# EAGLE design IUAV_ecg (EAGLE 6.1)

## Sheet 1 of 5: Info
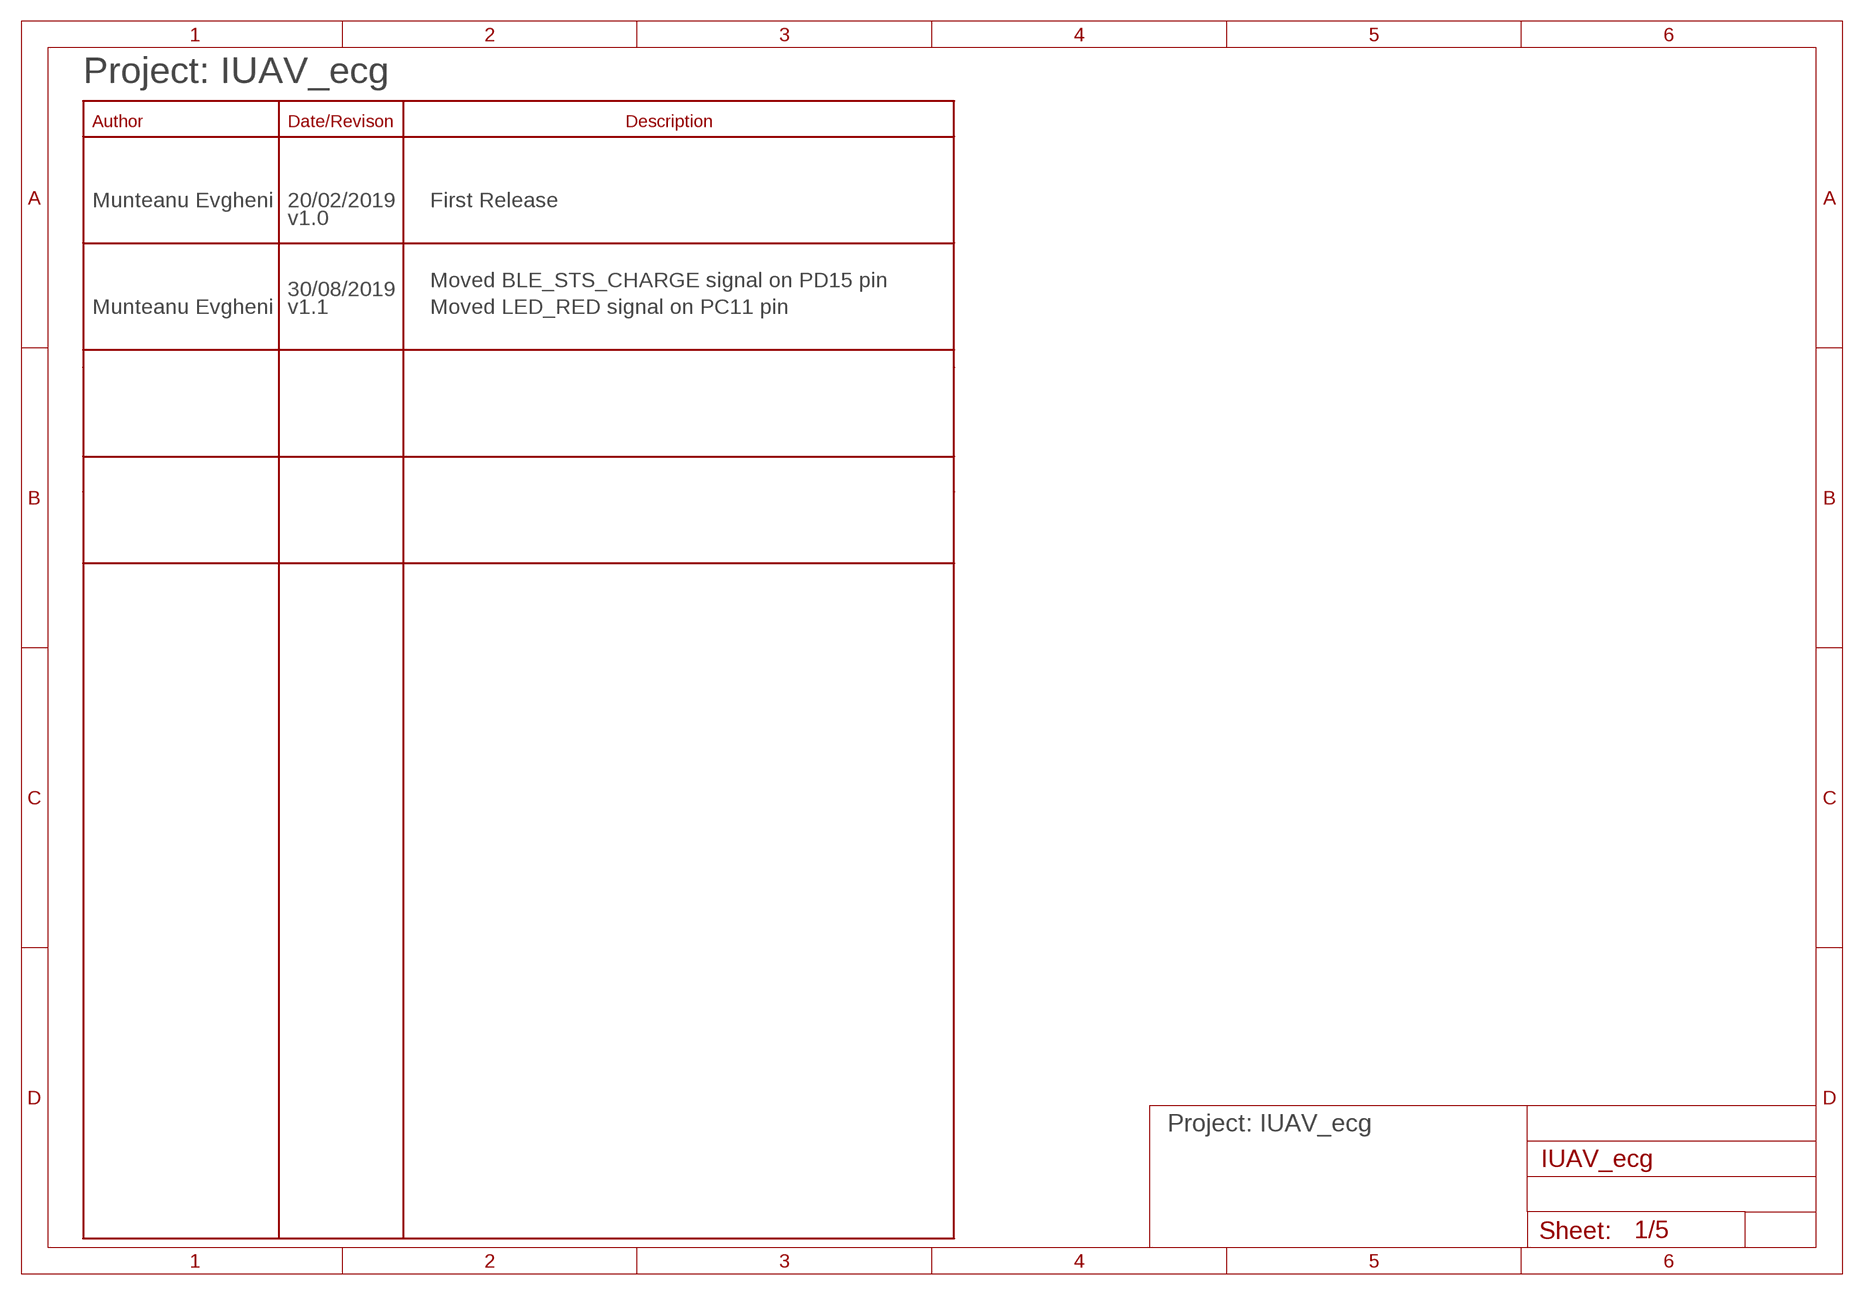
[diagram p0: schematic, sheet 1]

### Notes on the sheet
- Project: IUAV_ecg
- Munteanu Evgheni | 20/02/2019 | First Release
- v1.0
- Moved BLE_STS_CHARGE signal on PD15 pin
- 30/08/2019
- Munteanu Evgheni | v1.1 | Moved LED_RED signal on PC11 pin
- Project: IUAV_ecg

## Sheet 2 of 5: Power Management
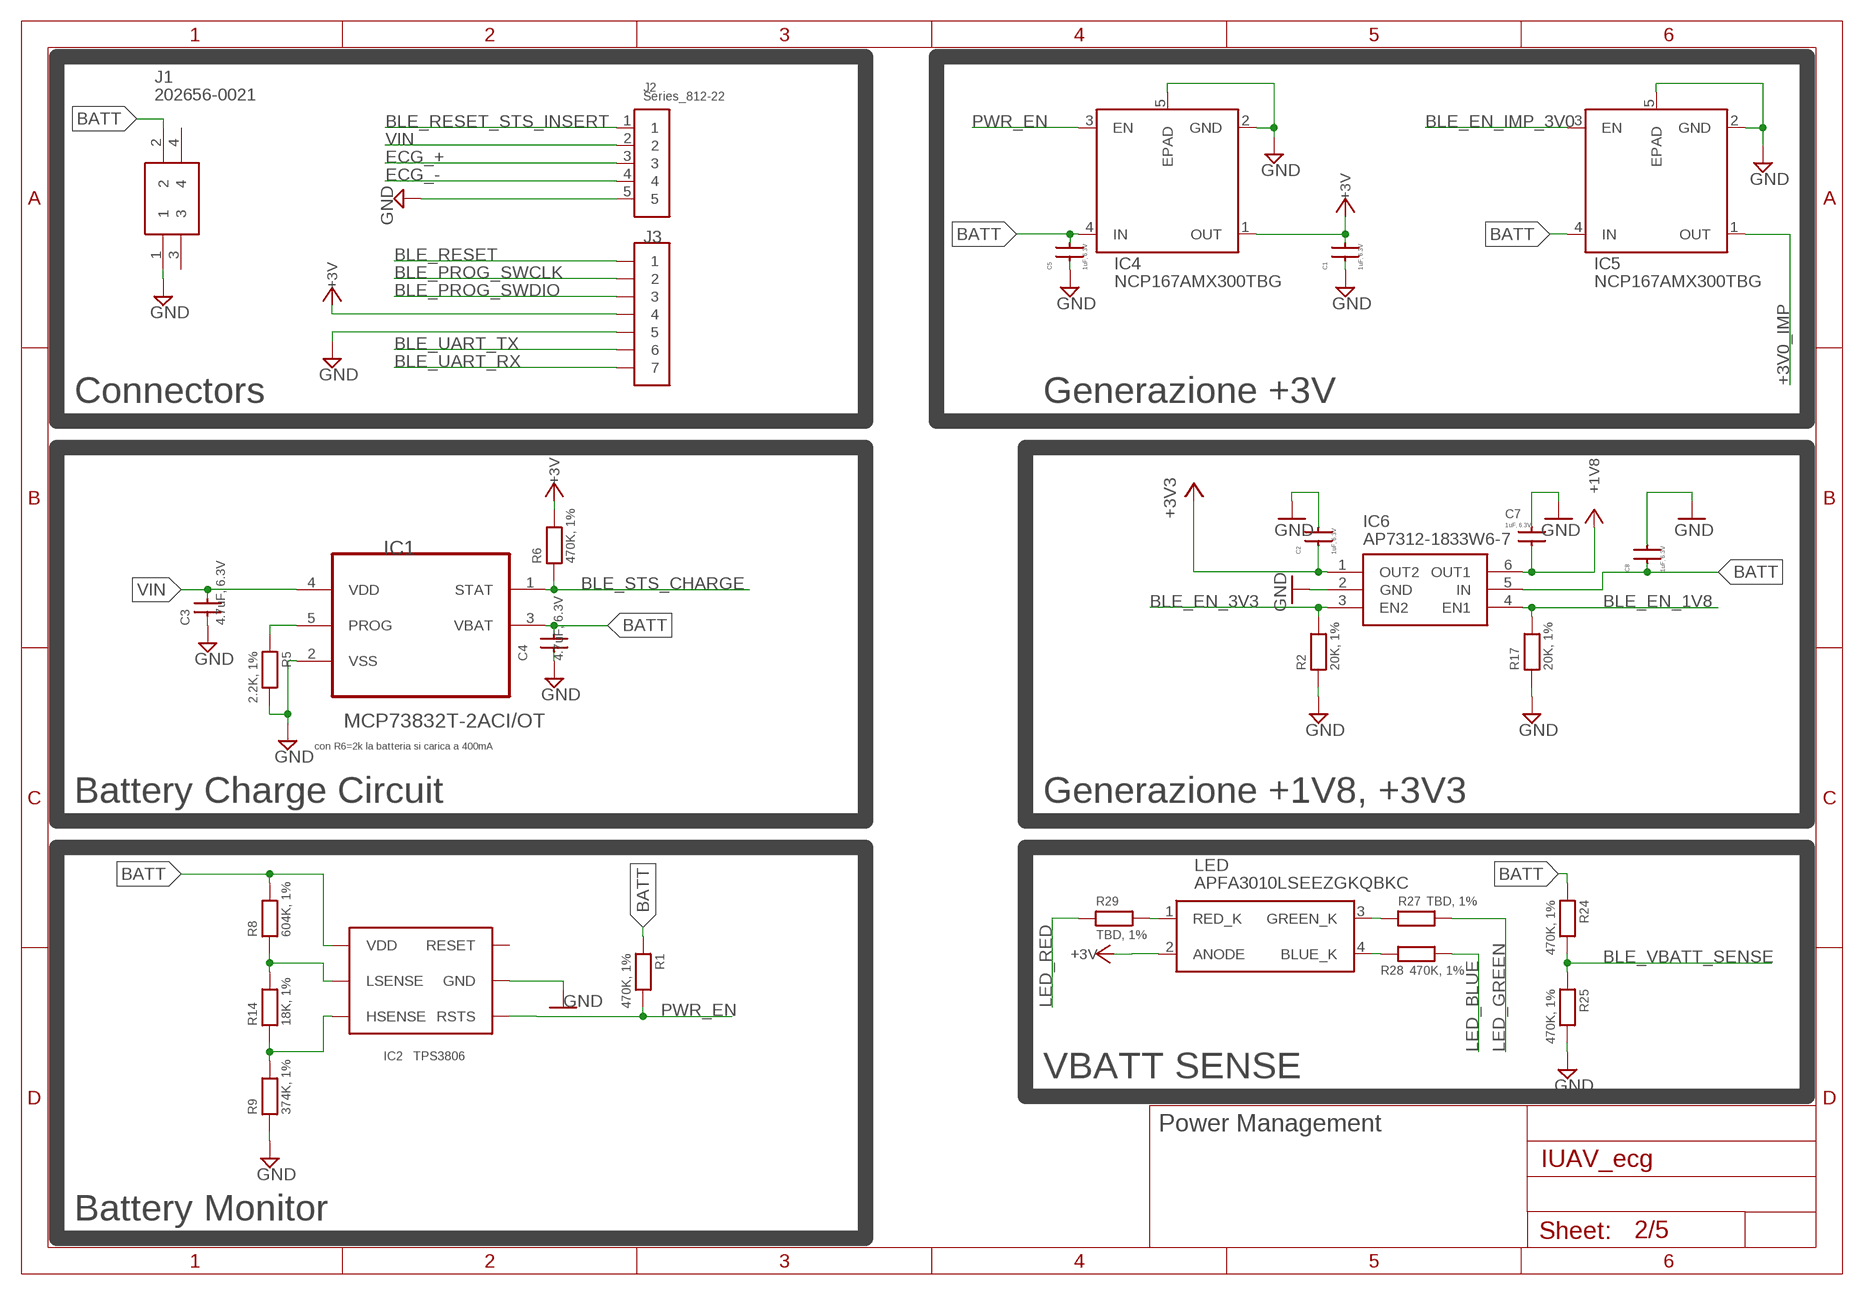
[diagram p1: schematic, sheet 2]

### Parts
C1  1uF, 6.3V  C0402  [R0402]
C2  1uF, 6.3V  C0402  [R0402]
C3  4.7uF, 6.3V  C0402  [R0402]
C4  4.7uF, 6.3V  C0402  [R0402]
C5  1uF, 6.3V  C0402  [R0402]
C7  1uF, 6.3V  C0402  [R0402]
C8  1uF, 6.3V  C0402  [R0402]
IC1  MCP73832T-2ACI/OT  MCP73831T-2ACI/OT  [SOT95P280X145-5N]
IC2  TPS3806  [SOT23_6_DBV]
IC4  NCP167AMX300TBG  NCP167  [NCP167]
IC5  NCP167AMX300TBG  NCP167  [NCP167]
IC6  AP7312-1833W6-7  [SOT95P285X145-6N]
J1  202656-0021  [2026560021]
J2  Series_812-22  CONNECTOR_MOLLA_2.54_5P  [CONNETTORE_MOLLA_2.54_5P]
J3  PINS_PROG_1.27MM_7P  [PINS_GENERIC_1.27_7P]
LED  APFA3010LSEEZGKQBKC  [KPFA-3010RGBC-11]
R1  470K, 1%  R0402  [R0402]
R2  20K, 1%  R0402  [R0402]
R5  2.2K, 1%  R0402  [R0402]
R6  470K, 1%  R0402  [R0402]
R8  604K, 1%  R0402  [R0402]
R9  374K, 1%  R0402  [R0402]
R14  18K, 1%  R0402  [R0402]
R17  20K, 1%  R0402  [R0402]
R24  470K, 1%  R0402  [R0402]
R25  470K, 1%  R0402  [R0402]
R27  TBD, 1%  R0402  [R0402]
R28  470K, 1%  R0402  [R0402]
R29  TBD, 1%  R0402  [R0402]

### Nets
+1V8: C7.P$1 IC6.6(OUT1) ; also sheet 5
+3V: C1.P$2 IC4.1(OUT) J3.4 LED.2(ANODE) R6.P$2 ; also sheet 3,5
+3V0_IMP: IC5.1(OUT) ; also sheet 4
+3V3: C2.P$1 IC6.1(OUT2) ; also sheet 5
BATT: C4.P$2 C5.P$2 C8.P$1 IC1.3(VBAT) IC2.P$4(VDD) IC4.4(IN) IC5.4(IN) IC6.5(IN) J1.2 R1.P$1 R8.P$2 R24.P$1
BLE_EN_1V8: IC6.4(EN1) R17.P$2 ; also sheet 3
BLE_EN_3V3: IC6.3(EN2) R2.P$2 ; also sheet 3
BLE_EN_IMP_3V0: IC5.3(EN) ; also sheet 3
BLE_PROG_SWCLK: J3.2 ; also sheet 3
BLE_PROG_SWDIO: J3.3 ; also sheet 3
BLE_RESET: J3.1 ; also sheet 3
BLE_RESET_STS_INSERT: J2.1 ; also sheet 3
BLE_STS_CHARGE: IC1.1(STAT) R6.P$1 ; also sheet 3
BLE_UART_RX: J3.7 ; also sheet 3
BLE_UART_TX: J3.6 ; also sheet 3
BLE_VBATT_SENSE: R24.P$2 R25.P$1 ; also sheet 3
ECG_+: J2.3 ; also sheet 5
ECG_-: J2.4 ; also sheet 5
GND: C1.P$1 C2.P$2 C3.P$1 C4.P$1 C5.P$1 C7.P$2 C8.P$2 IC1.2(VSS) IC2.P$2(GND) IC4.2(GND) IC4.5(EPAD) IC5.2(GND) IC5.5(EPAD) IC6.2(GND) J1.1 J2.5 J3.5 R2.P$1 R5.P$2 R9.P$1 R17.P$1 R25.P$2 ; also sheet 3,4,5
LED_BLUE: R28.P$1 ; also sheet 3
LED_GREEN: R27.P$2 ; also sheet 3
LED_RED: R29.P$1 ; also sheet 3
N$9: IC1.5(PROG) R5.P$1
N$11: IC2.P$5(LSENSE) R8.P$1 R14.P$2
N$13: IC2.P$6(HSENSE) R9.P$2 R14.P$1
N$17: LED.1(RED_K) R29.P$2
N$18: LED.4(BLUE_K) R28.P$2
N$19: LED.3(GREEN_K) R27.P$1
PWR_EN: IC2.P$1(RSTS) IC4.3(EN) R1.P$2
VIN: C3.P$2 IC1.4(VDD) J2.2
Unconnected: IC2.P$3(RESET) J1.3 J1.4

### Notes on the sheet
- Connectors | Generazione +3V
- con R6=2k la batteria si carica a 400mA
- Battery Charge Circuit | Generazione +1V8, +3V3
- VBATT SENSE
- Power Management
- Battery Monitor

## Sheet 3 of 5: Bluetooth
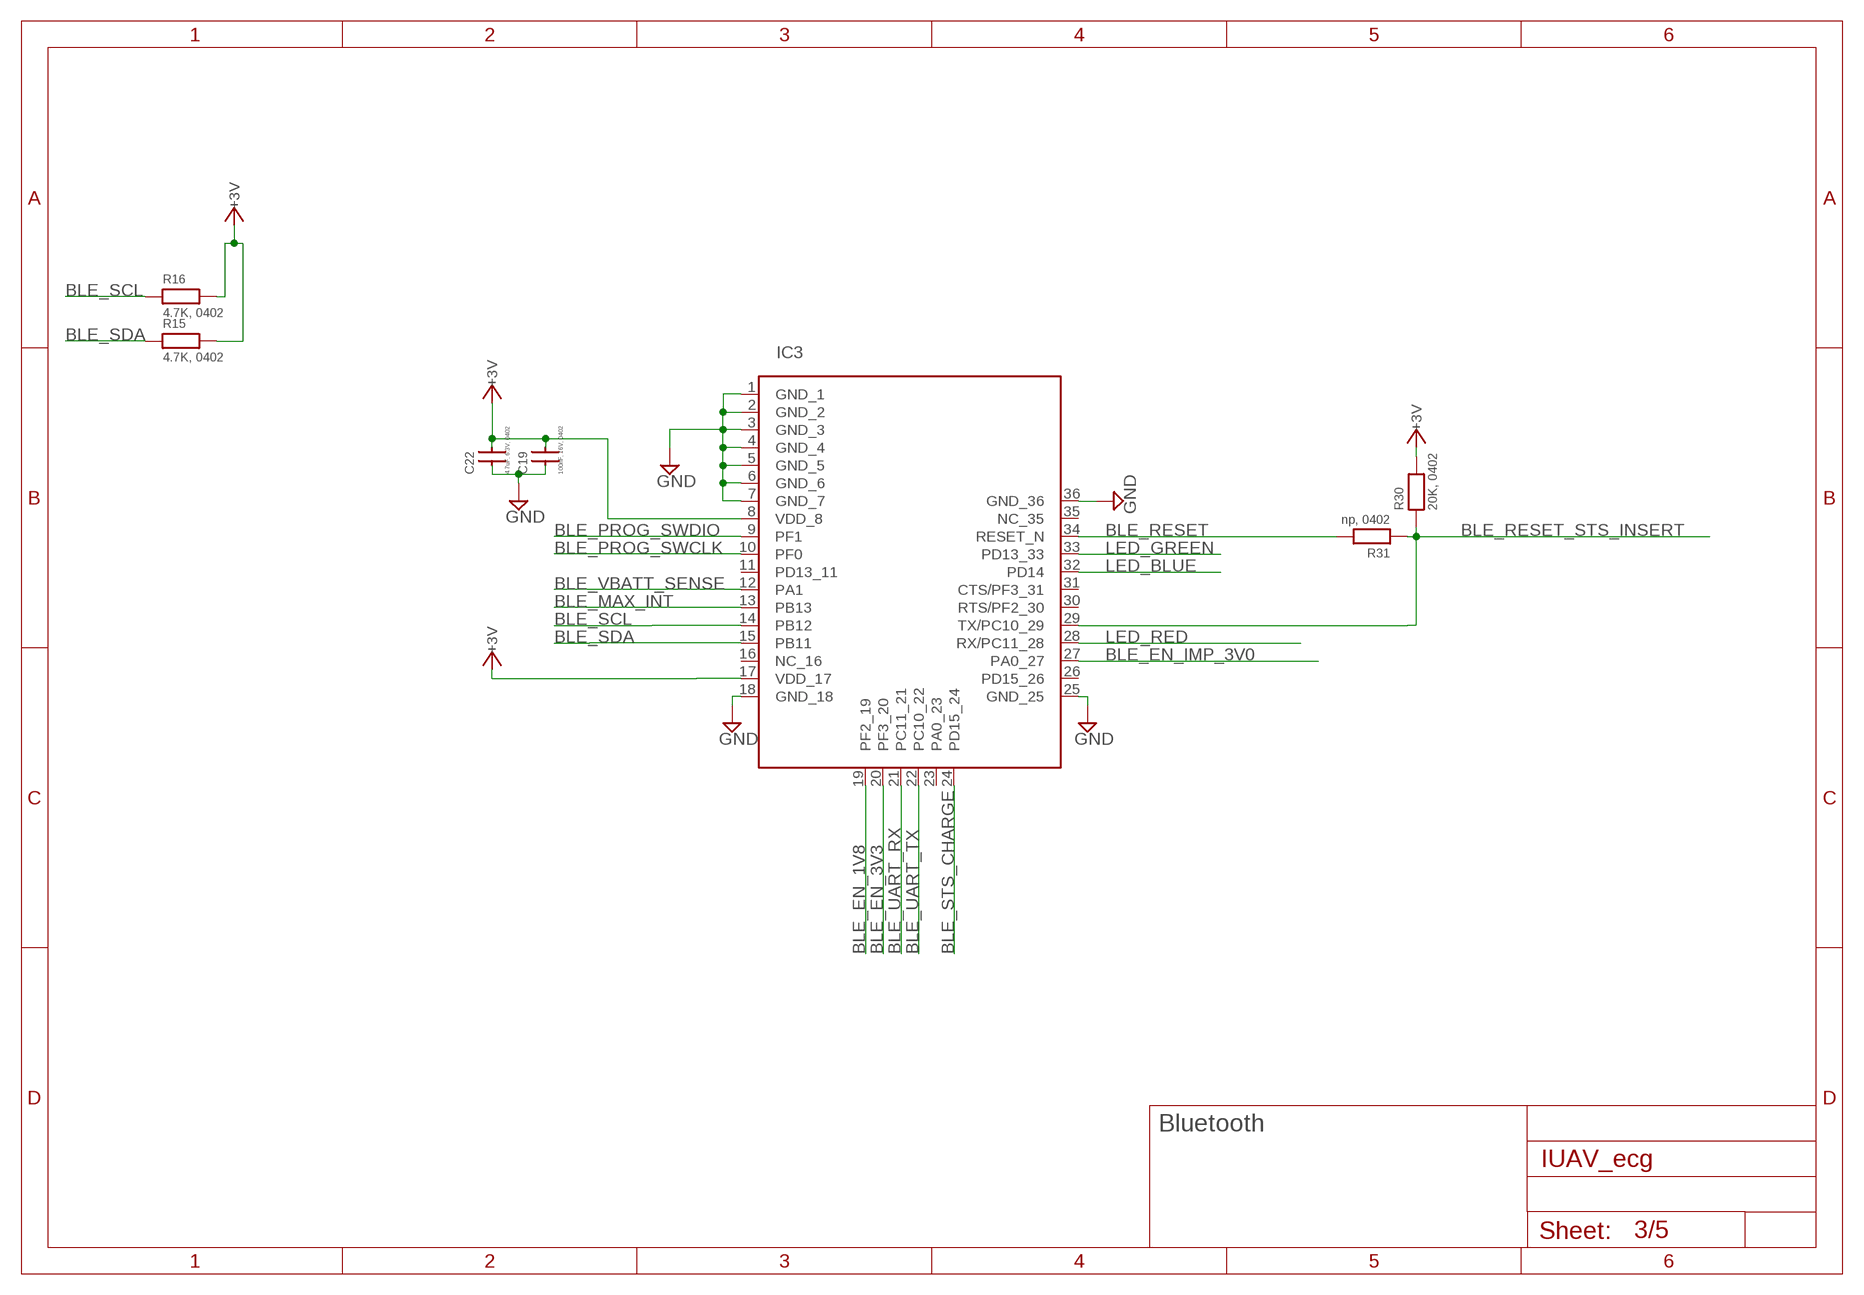
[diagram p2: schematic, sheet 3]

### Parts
C19  100nF, 16V, 0402  C0402  [R0402]
C22  4.7uF, 6.3V, 0402  C0402  [R0402]
IC3  BGM113  [BGM113]
R15  4.7K, 0402  R0402  [R0402]
R16  4.7K, 0402  R0402  [R0402]
R30  20K, 0402  R0402  [R0402]
R31  np, 0402  R0402  [R0402]

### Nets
+3V: C19.P$2 C22.P$2 IC3.8(VDD_8) IC3.17(VDD_17) R15.P$2 R16.P$2 R30.P$2 ; also sheet 2,5
BLE_EN_1V8: IC3.19(PF2_19) ; also sheet 2
BLE_EN_3V3: IC3.20(PF3_20) ; also sheet 2
BLE_EN_IMP_3V0: IC3.27(PA0_27) ; also sheet 2
BLE_MAX_INT: IC3.13(PB13) ; also sheet 5
BLE_PROG_SWCLK: IC3.10(PF0) ; also sheet 2
BLE_PROG_SWDIO: IC3.9(PF1) ; also sheet 2
BLE_RESET: IC3.34(RESET_N) R31.P$2 ; also sheet 2
BLE_RESET_STS_INSERT: IC3.29(TX/PC10_29) R30.P$1 R31.P$1 ; also sheet 2
BLE_SCL: IC3.14(PB12) R16.P$1 ; also sheet 4,5
BLE_SDA: IC3.15(PB11) R15.P$1 ; also sheet 4,5
BLE_STS_CHARGE: IC3.24(PD15_24) ; also sheet 2
BLE_UART_RX: IC3.21(PC11_21) ; also sheet 2
BLE_UART_TX: IC3.22(PC10_22) ; also sheet 2
BLE_VBATT_SENSE: IC3.12(PA1) ; also sheet 2
GND: C19.P$1 C22.P$1 IC3.1(GND_1) IC3.2(GND_2) IC3.3(GND_3) IC3.4(GND_4) IC3.5(GND_5) IC3.6(GND_6) IC3.7(GND_7) IC3.18(GND_18) IC3.25(GND_25) IC3.36(GND_36) ; also sheet 2,4,5
LED_BLUE: IC3.32(PD14) ; also sheet 2
LED_GREEN: IC3.33(PD13_33) ; also sheet 2
LED_RED: IC3.28(RX/PC11_28) ; also sheet 2
Unconnected: IC3.11(PD13_11) IC3.16(NC_16) IC3.23(PA0_23) IC3.26(PD15_26) IC3.30(RTS/PF2_30) IC3.31(CTS/PF3_31) IC3.35(NC_35)

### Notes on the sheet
- Bluetooth

## Sheet 4 of 5: Sensore Impedenza
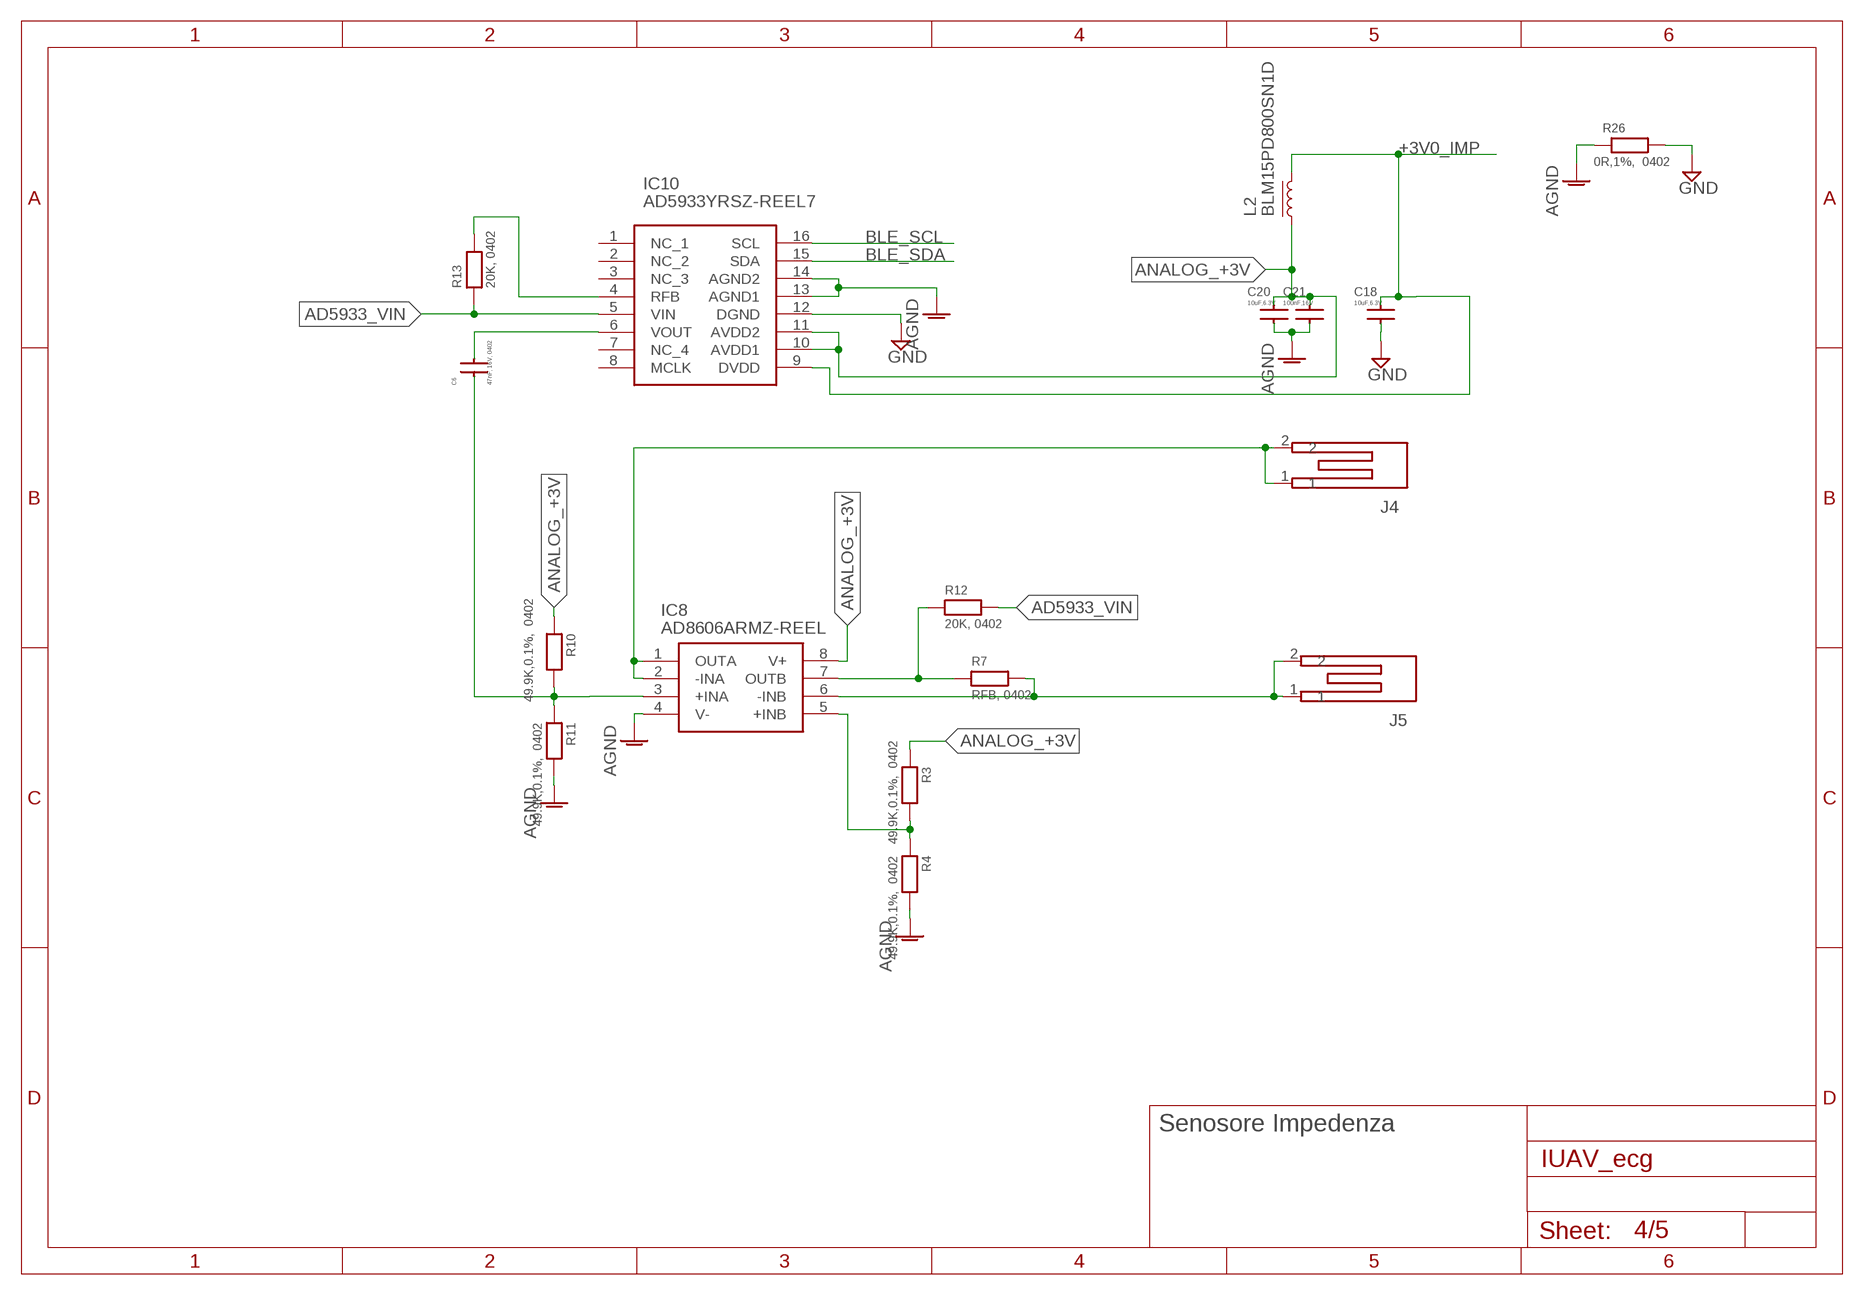
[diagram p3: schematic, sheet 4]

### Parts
C6  47nF, 16V, 0402  C0402  [R0402]
C18  10uF,6.3V  C0402  [R0402]
C20  10uF,6.3V  C0402  [R0402]
C21  100nF,16V  C0402  [R0402]
IC8  AD8606ARMZ-REEL  [SOP65P490X110-8N]
IC10  AD5933YRSZ-REEL7  [SOP65P780X200-16N]
J4  CONTACT_2040852-1  [CONTACT_2040852-1]
J5  CONTACT_2040852-1  [CONTACT_2040852-1]
L2  BLM15PD800SN1D  INDUTTORE_FILTRO  [SMD_0402]
R3  49.9K,0.1%, 0402  R0402  [R0402]
R4  49.9K,0.1%, 0402  R0402  [R0402]
R7  RFB, 0402  R0402  [R0402]
R10  49.9K,0.1%, 0402  R0402  [R0402]
R11  49.9K,0.1%, 0402  R0402  [R0402]
R12  20K, 0402  R0402  [R0402]
R13  20K, 0402  R0402  [R0402]
R26  0R,1%, 0402  R0402  [R0402]

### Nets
+3V0_IMP: C18.P$2 IC10.9(DVDD) L2.P$2 ; also sheet 2
AD5933_VIN: IC10.5(VIN) R12.P$2 R13.P$1
AGND: C20.P$1 C21.P$1 IC8.4(V-) IC10.13(AGND1) IC10.14(AGND2) R4.P$2 R11.P$2 R26.P$1
ANALOG_+3V: C20.P$2 C21.P$2 IC8.8(V+) IC10.10(AVDD1) IC10.11(AVDD2) L2.P$1 R3.P$1 R10.P$1
BLE_SCL: IC10.16(SCL) ; also sheet 3,5
BLE_SDA: IC10.15(SDA) ; also sheet 3,5
GND: C18.P$1 IC10.12(DGND) R26.P$2 ; also sheet 2,3,5
N$4: IC8.5(+INB) R3.P$2 R4.P$1
N$5: IC8.7(OUTB) R7.P$1 R12.P$1
N$6: IC8.6(-INB) J5.1 J5.2 R7.P$2
N$8: C6.P$2 IC10.6(VOUT)
N$10: C6.P$1 IC8.3(+INA) R10.P$2 R11.P$1
N$14: IC8.1(OUTA) IC8.2(-INA) J4.1 J4.2
N$16: IC10.4(RFB) R13.P$2
Unconnected: IC10.1(NC_1) IC10.2(NC_2) IC10.3(NC_3) IC10.7(NC_4) IC10.8(MCLK)

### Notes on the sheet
- Senosore Impedenza

## Sheet 5 of 5: Sensore ECG
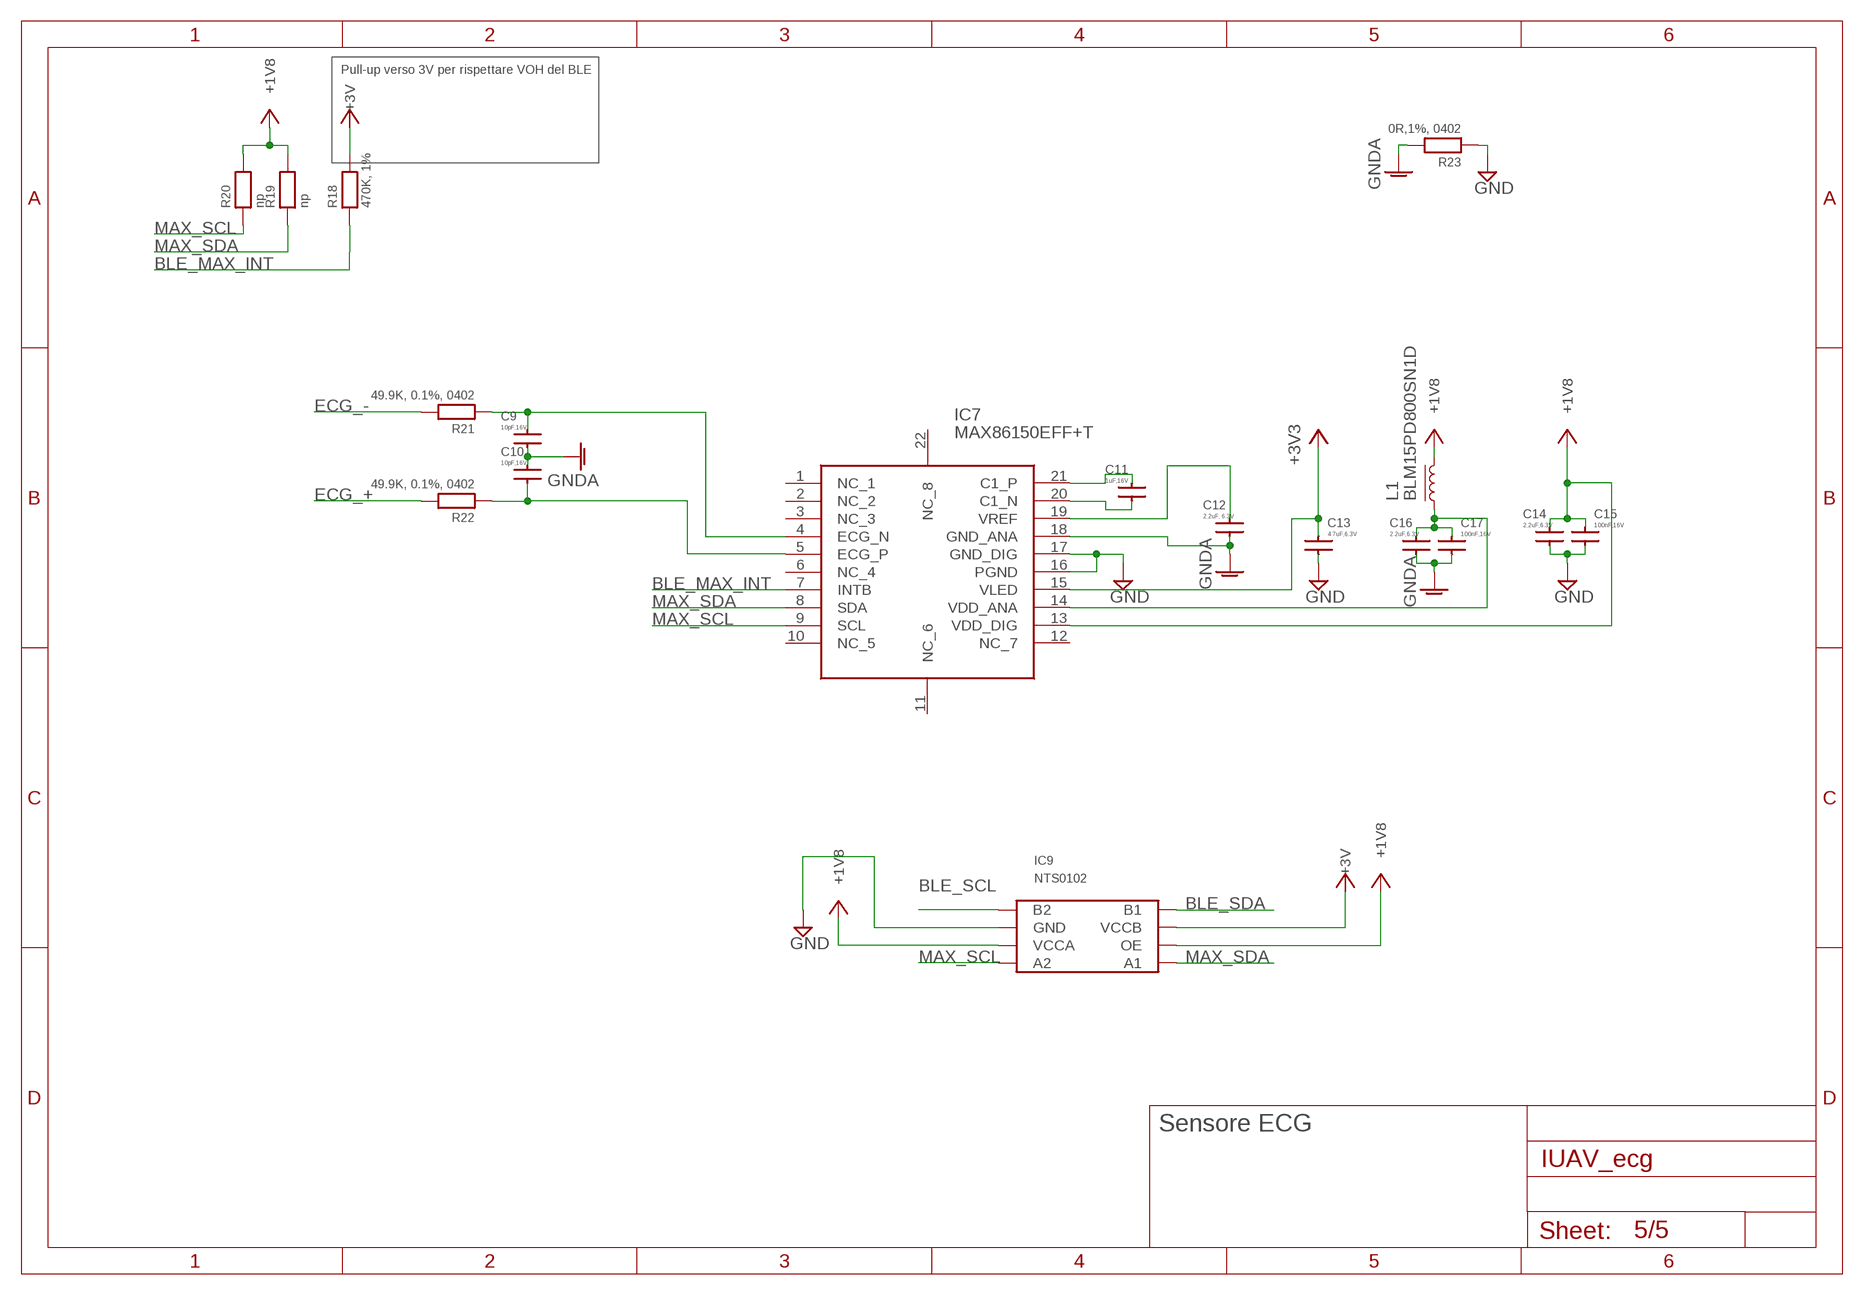
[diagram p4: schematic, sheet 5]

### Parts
C9  10pF,16V  C0402  [R0402]
C10  10pF,16V  C0402  [R0402]
C11  1uF,16V  C0402  [R0402]
C12  2.2uF, 6.3V  C0402  [R0402]
C13  4.7uF,6.3V  C0402  [R0402]
C14  2.2uF,6.3V  C0402  [R0402]
C15  100nF,16V  C0402  [R0402]
C16  2.2uF,6.3V  C0402  [R0402]
C17  100nF,16V  C0402  [R0402]
IC7  MAX86150EFF+T  [MAX86150EFFT]
IC9  NTS0102  [SOT996-2]
L1  BLM15PD800SN1D  INDUTTORE_FILTRO  [SMD_0402]
R18  470K, 1%  R0402  [R0402]
R19  np  R0402  [R0402]
R20  np  R0402  [R0402]
R21  49.9K, 0.1%, 0402  R0402  [R0402]
R22  49.9K, 0.1%, 0402  R0402  [R0402]
R23  0R,1%, 0402  R0402  [R0402]

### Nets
+1V8: C14.P$2 C15.P$2 IC7.13(VDD_DIG) IC9.3(VCCA) IC9.6(OE) L1.P$2 R19.P$2 R20.P$2 ; also sheet 2
+3V: IC9.7(VCCB) R18.P$2 ; also sheet 2,3
+3V3: C13.P$2 IC7.15(VLED) ; also sheet 2
BLE_MAX_INT: IC7.7(INTB) R18.P$1 ; also sheet 3
BLE_SCL: IC9.1(B2) ; also sheet 3,4
BLE_SDA: IC9.8(B1) ; also sheet 3,4
ECG_+: R22.P$2 ; also sheet 2
ECG_-: R21.P$2 ; also sheet 2
GND: C13.P$1 C14.P$1 C15.P$1 IC7.16(PGND) IC7.17(GND_DIG) IC9.2(GND) R23.P$1 ; also sheet 2,3,4
GNDA: C9.P$1 C10.P$2 C12.P$1 C16.P$1 C17.P$1 IC7.18(GND_ANA) R23.P$2
MAX_SCL: IC7.9(SCL) IC9.4(A2) R20.P$1
MAX_SDA: IC7.8(SDA) IC9.5(A1) R19.P$1
N$1: C9.P$2 IC7.4(ECG_N) R21.P$1
N$2: C11.P$2 IC7.21(C1_P)
N$3: C10.P$1 IC7.5(ECG_P) R22.P$1
N$7: C11.P$1 IC7.20(C1_N)
N$12: C12.P$2 IC7.19(VREF)
N$15: C16.P$2 C17.P$2 IC7.14(VDD_ANA) L1.P$1
Unconnected: IC7.1(NC_1) IC7.2(NC_2) IC7.3(NC_3) IC7.6(NC_4) IC7.10(NC_5) IC7.11(NC_6) IC7.12(NC_7) IC7.22(NC_8)

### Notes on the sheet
- Pull-up verso 3V per rispettare VOH del BLE
- Sensore ECG

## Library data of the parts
C1-C22 = VIBRAM_LIB:C0402
IC1 = vibram:MCP73831T-2ACI/OT: Charge Management Controller; MPN: MCP73831T-2ACI/OT; OC_FARNELL: 1332158; OC_NEWARK: 56K7045; PACKAGE: SOT-5; SUPPLIER: Microchip
IC2 = VIBRAM_LIB:TPS3806
IC3 = RELab_ElectronicLibrary:BGM113
IC4 IC5 = RELab_ElectronicLibrary:NCP167
IC6 = SamacSys_Parts:AP7312-1833W6-7: LDO,Regulator,Pos,reg,3.3V,0.15A,SOT26 DiodesZetex AP7312-1833W6-7, Dual LDO Voltage Regulator, 150mA, 1.8 V, 3.3 V /-2%, 6-Pin SOT-26 Source: Datasheet; DESCRIPTION: LDO,Regulator,Pos,reg,3.3V,0.15A,SOT26 DiodesZetex AP7312-1833W6-7, Dual LDO Voltage Regulator, 150mA, 1.8 V, 3.3 V /-2%, 6-Pin SOT-26; HEIGHT: 1.45mm; MANUFACTURER_NAME: Diodes Inc.; MANUFACTURER_PART_NUMBER: AP7312-1833W6-7; MOUSER_PART_NUMBER: 621-AP7312-1833W6-7; MOUSER_PRICE-STOCK: https://www.mouser.com/Search/Refine.aspx?Keyword=621-AP7312-1833W6-7
IC7 = SamacSys_Parts:MAX86150EFF+T: Biometric Sensors Pulse Oximetry/Heart Rate Bio Sensor Source: Datasheet; DESCRIPTION: Biometric Sensors Pulse Oximetry/Heart Rate Bio Sensor; HEIGHT: 1.4mm; MANUFACTURER_NAME: Maxim Integrated; MANUFACTURER_PART_NUMBER: MAX86150EFF+T; MOUSER_PART_NUMBER: 700-MAX86150EFF+T; MOUSER_PRICE-STOCK: https://www.mouser.com/Search/Refine.aspx?Keyword=700-MAX86150EFF%2BT
IC8 = SamacSys_Parts:AD8606ARMZ-REEL: Precision, Low Noise, CMOS, Rail-to-Rail,%D Input/Output Operational Amplifiers Source: Datasheet; DESCRIPTION: Precision, Low Noise, CMOS, Rail-to-Rail,%D Input/Output Operational Amplifiers; HEIGHT: 1.1mm; MANUFACTURER_NAME: Analog Devices; MANUFACTURER_PART_NUMBER: AD8606ARMZ-REEL; MOUSER_PART_NUMBER: 584-AD8606ARMZ-R; MOUSER_PRICE-STOCK: https://www.mouser.com/Search/Refine.aspx?Keyword=584-AD8606ARMZ-R
IC9 = RELab_ElectronicLibrary:NTS0102
IC10 = SamacSys_Parts:AD5933YRSZ-REEL7: Data Acquisition ADCs/DACs - Specialized IC 12bit 1 MSPS Impedance Cnvtr Source: Datasheet; DESCRIPTION: Data Acquisition ADCs/DACs - Specialized IC 12bit 1 MSPS Impedance Cnvtr; HEIGHT: 2mm; MANUFACTURER_NAME: Analog Devices; MANUFACTURER_PART_NUMBER: AD5933YRSZ-REEL7; MOUSER_PART_NUMBER: 584-AD5933YRSZ-R7; MOUSER_PRICE-STOCK: https://www.mouser.com/Search/Refine.aspx?Keyword=584-AD5933YRSZ-R7
J1 = SamacSys_Parts:202656-0021: MOLEX - 202656-0021 - PLUG HOUSING, 2POS, NYLON, BLACK Source: Datasheet; DESCRIPTION: MOLEX - 202656-0021 - PLUG HOUSING, 2POS, NYLON, BLACK; HEIGHT: 1mm; MANUFACTURER_NAME: Molex; MANUFACTURER_PART_NUMBER: 202656-0021; MOUSER_PART_NUMBER: 538-202656-0021; MOUSER_PRICE-STOCK: https://www.mouser.com/Search/Refine.aspx?Keyword=538-202656-0021
J2 = RELab_ElectronicLibrary:CONNECTOR_MOLLA_2.54_5P
J3 = RELab_ElectronicLibrary:PINS_PROG_1.27MM_7P
J4 J5 = RELab_ElectronicLibrary:CONTACT_2040852-1
L1 L2 = RELab_ElectronicLibrary:INDUTTORE_FILTRO
LED = SamacSys_Parts:APFA3010LSEEZGKQBKC: 3.0x1.0mm RIGHT ANGLE SMD CHIP LED LAMP Source: Datasheet; DESCRIPTION: 3.0x1.0mm RIGHT ANGLE SMD CHIP LED LAMP; HEIGHT: mm; MANUFACTURER_NAME: Kingbright; MANUFACTURER_PART_NUMBER: APFA3010LSEEZGKQBKC; MOUSER_PART_NUMBER: 604-APFA3010LSEEZGKQ; MOUSER_PRICE-STOCK: https://www.mouser.com/Search/Refine.aspx?Keyword=604-APFA3010LSEEZGKQ
R1-R31 = VIBRAM_LIB:R0402

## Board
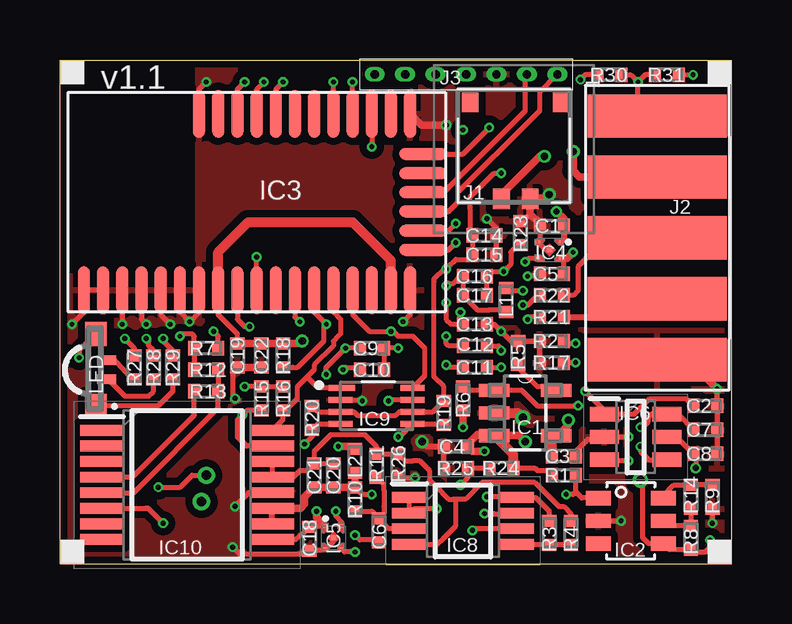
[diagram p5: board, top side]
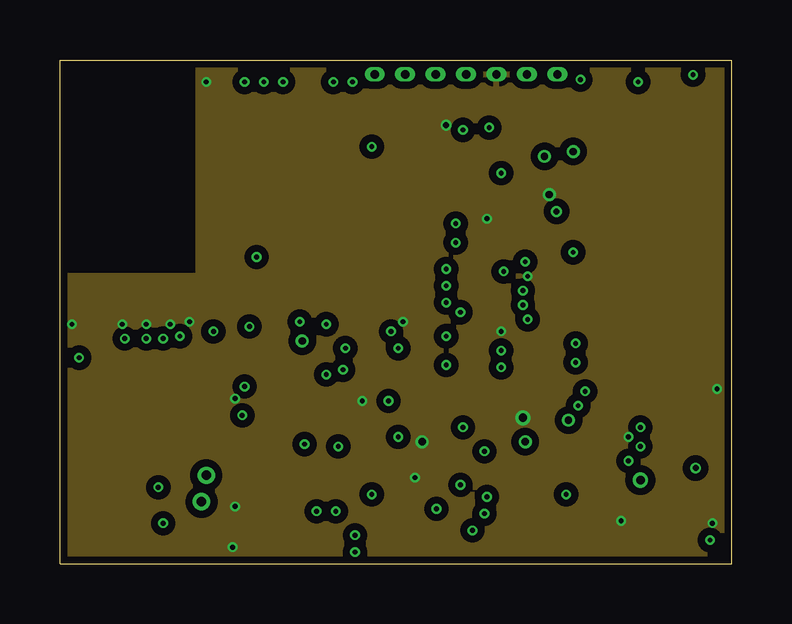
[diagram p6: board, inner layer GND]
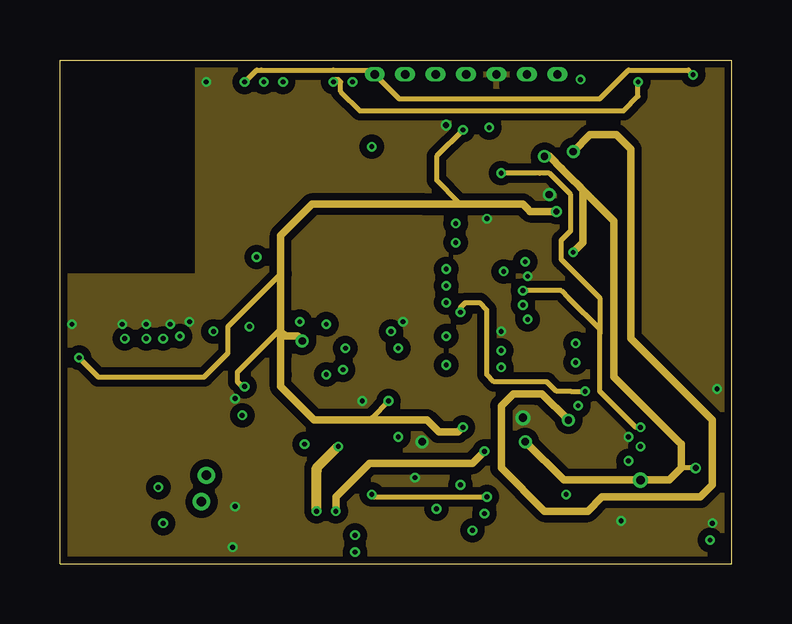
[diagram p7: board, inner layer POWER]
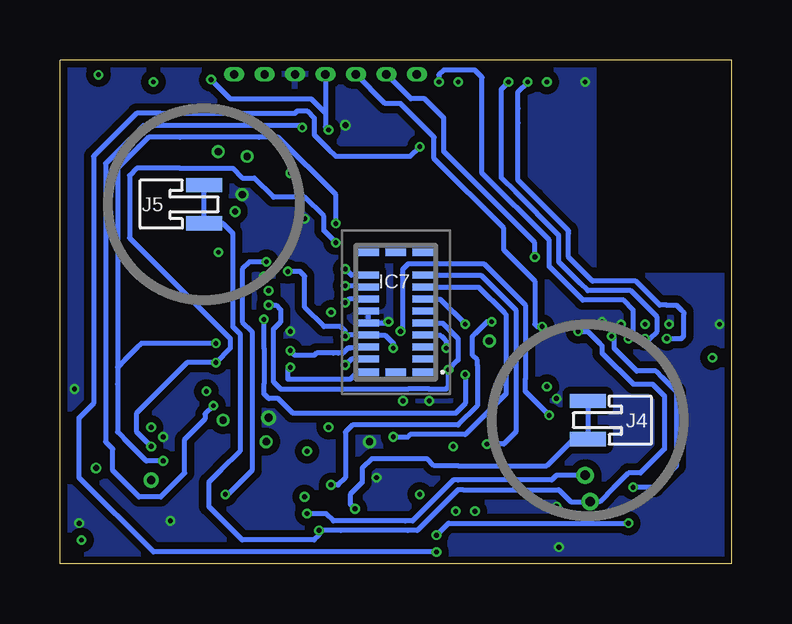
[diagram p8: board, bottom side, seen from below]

Size 28 x 21 mm. Coordinates in mm from the lower left corner, seen from the top.
Outline: 28,0 28,21 0,21 0,0 28,0
Copper layers (1+2*3+16): Top 0.035mm / dielectric 0.38mm / GND 0.035mm / dielectric 0.71mm / POWER 0.035mm / dielectric 0.38mm / Bottom 0.035mm
Design rules: minimum track width 0.2mm, minimum drill 0.2mm, track to track 0.2mm, track to pad 0.2mm, pad to pad 0.2mm, via to via 0.2mm, smd to smd 0.15mm, copper to edge 0.2mm, drill to drill 0.2mm, minimum pad ring 0.1mm, minimum via ring 0.1mm, stop-mask expansion 0.075mm, vias tented up to drill 12mil, thermal gap 0.2mm

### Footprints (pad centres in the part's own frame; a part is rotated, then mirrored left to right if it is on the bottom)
R0402 = smd 0.5 x 0.6: P$1 -0.5,0; P$2 0.5,0
SOT95P280X145-5N = smd 1.27 x 0.559: 1 -1.295,0.94; 2 -1.295,0; 3 -1.295,-0.94; 4 1.295,-0.94; 5 1.295,0.94
SOT23_6_DBV = smd 0.6 x 1.05: P$1 -0.95,-1.35; P$2 0,-1.35; P$3 0.95,-1.35; P$4 0.95,1.35; P$5 0,1.35; P$6 -0.95,1.35
BGM113 = smd 2 x 0.5: 1 -3.675,7.2; 2 -3.675,6.4; 3 -3.675,5.6; 4 -3.675,4.8; 5 -3.675,4; 6 -3.675,3.2; 7 -3.675,2.4; 8 -3.675,1.6; 9 -3.675,0.8; 10 -3.675,0; 11 -3.675,-0.8; 12 -3.675,-1.6; 13 -3.675,-2.4; 14 -3.675,-3.2; 15 -3.675,-4; 16 -3.675,-4.8; 17 -3.675,-5.6; 18 -3.675,-6.4; 25 3.675,-6.4; 26 3.675,-5.6; 27 3.675,-4.8; 28 3.675,-4; 29 3.675,-3.2; 30 3.675,-2.4; 31 3.675,-1.6; 32 3.675,-0.8; 33 3.675,0; 34 3.675,0.8; 35 3.675,1.6; 36 3.675,2.4 | smd 0.5 x 2: 19 -2,-6.95; 20 -1.2,-6.95; 21 -0.4,-6.95; 22 0.4,-6.95; 23 1.2,-6.95; 24 2,-6.95
NCP167 = smd 0.2 x 0.2: 1 -0.355,0.5; 2 -0.355,-0.5; 3 0.355,-0.5; 4 0.355,0.5; 5 0,0
SOT95P285X145-6N = smd 1.2 x 0.6: 1 -1.3,0.95; 2 -1.3,0; 3 -1.3,-0.95; 4 1.3,-0.95; 5 1.3,0; 6 1.3,0.95
MAX86150EFFT = smd 0.9 x 0.3: 1 -1.15,2.5; 2 -1.15,1.95; 3 -1.15,1.45; 4 -1.15,0.95; 5 -1.15,0.45; 6 -1.15,-0.05; 7 -1.15,-0.55; 8 -1.15,-1.05; 9 -1.15,-1.55; 10 -1.15,-2.5; 12 1.15,-2.5; 13 1.15,-1.55; 14 1.15,-1.05; 15 1.15,-0.55; 16 1.15,-0.05; 17 1.15,0.45; 18 1.15,0.95; 19 1.15,1.45; 20 1.15,1.95; 21 1.15,2.5 | smd 0.85 x 0.3: 11 0,-2.5; 22 0,2.5
SOP65P490X110-8N = smd 1.45 x 0.45: 1 -2.225,0.975; 2 -2.225,0.325; 3 -2.225,-0.325; 4 -2.225,-0.975; 5 2.225,-0.975; 6 2.225,-0.325; 7 2.225,0.325; 8 2.225,0.975
SOT996-2 = smd 0.25 x 1.1: 1 -0.75,-1.45 | smd 0.25 x 1: 2 -0.25,-1.5; 3 0.25,-1.5; 4 0.75,-1.5; 5 0.75,1.5; 6 0.25,1.5; 7 -0.25,1.5; 8 -0.75,1.5
SOP65P780X200-16N = smd 1.8 x 0.45: 1 -3.55,2.275; 2 -3.55,1.625; 3 -3.55,0.975; 4 -3.55,0.325; 5 -3.55,-0.325; 6 -3.55,-0.975; 7 -3.55,-1.625; 8 -3.55,-2.275; 9 3.55,-2.275; 10 3.55,-1.625; 11 3.55,-0.975; 12 3.55,-0.325; 13 3.55,0.325; 14 3.55,0.975; 15 3.55,1.625; 16 3.55,2.275
2026560021 = smd 0.7 x 0.85: 1 -0.6,2.072; 2 0.6,2.072 | smd 0.7 x 0.8: 3 -1.9,-1.953; 4 1.9,-1.953
CONNETTORE_MOLLA_2.54_5P = smd 1.8 x 5.8: 1 -5.08,0; 2 -2.54,0; 3 0,0; 4 2.54,0; 5 5.08,0
PINS_GENERIC_1.27_7P = drill 0.35 pad 0.6 long: 1 -3.81,0; 2 -2.54,0; 3 -1.27,0; 4 0,0; 5 1.27,0; 6 2.54,0; 7 3.81,0
CONTACT_2040852-1 = smd 1.5 x 0.6: 1 0,0.8; 2 0,-0.8
SMD_0402 = smd 0.5 x 0.6: P$1 -0.5,0; P$2 0.5,0
KPFA-3010RGBC-11 = smd 1 x 0.9: 1 1.5,-0.2; 2 -1.5,-0.2 | smd 0.4 x 0.8: 3 -0.4,0.25; 4 0.4,0.25

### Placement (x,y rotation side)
C1  20.5,14.1 0 top
C2  26.9,6.6 0 top
C3  21,4.5 180 top
C4  16.5,4.9 0 top
C5  20.5,12.1 0 top
C6  13.3,1.4 270 top
C7  26.9,5.6 0 top
C8  26.9,4.6 0 top
C9  13,9 180 top
C10  13,8.1 0 top
C11  17.3,8.2 0 top
C12  17.3,9.1 0 top
C13  17.3,10 180 top
C14  17.7,13.7 180 top
C15  17.7,12.9 180 top
C16  17.3,12 180 top
C17  17.3,11.2 180 top
C18  10.4,1.05 90 top
C19  7.4,8.7 90 top
C20  11.4,3.7 270 top
C21  10.6,3.7 270 top
C22  8.4,8.7 90 top
IC1  19.4,6.3 0 top
IC2  23.8,1.8 270 top
IC3  8.2,15.1 90 top
IC4  20.4,13.1 270 top
IC5  11.4,1.1 0 top
IC6  24,5.3 0 top
IC7  14,10.5 180 bottom
IC8  16.8,1.8 0 top
IC9  13.2,6.6 270 top
IC10  5.3,3.3 0 top
J1  19,17.3 180 top
J2  24.9,13.6 270 top
J3  16.93,20.42 0 top
J4  6,6 180 bottom
J5  22,15 0 bottom
L1  18.6,11 90 top
L2  12.3,4.3 90 top
LED  1.7,8.1 270 top
R1  21,3.7 0 top
R2  20.5,9.3 0 top
R3  20.4,1.3 270 top
R4  21.3,1.3 90 top
R5  19.1,8.8 90 top
R6  16.8,6.9 270 top
R7  6.1,9 0 top
R8  26.3,1.1 270 top
R9  27.2,2.8 90 top
R10  12.3,2.7 270 top
R11  13.2,4.1 90 top
R12  6.1,8.1 0 top
R13  6.1,7.2 180 top
R14  26.3,2.8 270 top
R15  8.4,6.9 90 top
R16  9.3,6.9 90 top
R17  20.5,8.4 0 top
R18  9.3,8.7 90 top
R19  16,6.3 90 top
R20  10.5,6.1 90 top
R21  20.5,10.3 0 top
R22  20.5,11.2 0 top
R23  19.2,13.8 270 top
R24  18.4,4 180 top
R25  16.5,4 180 top
R26  14.1,4.1 270 top
R27  3.1,8.2 90 top
R28  3.9,8.2 270 top
R29  4.7,8.2 270 top
R30  22.9,20.4 180 top
R31  25.3,20.4 0 top

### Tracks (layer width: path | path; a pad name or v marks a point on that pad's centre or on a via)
+1V8  (via drill 0.2)
  Top 0.2: C7.P$1 25.75,6.25 IC6.6 24.65,6.25 24.5,6.1 24.5,5.9 24.3,5.7 v24.2,5.7 | L1.P$2 18.7,11.4 v19.3,11.4 | R20.P$2 10.75,6.35 IC9.3 12.25,6.35 12.4,6.2 14,6.2 14.1,6.3 14.15,6.35 IC9.6 15.2,6.35 15.55,6.35 R19.P$2 16,7.4 15.6,7.8 15.6,11.8 15.6,11.9 16,12.3 v16.1,12.3 16.3,12.5 16.4,12.6 16.5,12.7 17,12.7 C15.P$2 C14.P$2 17.1,13.8 17.1,14.8 17.1,14.9 17.1,15.3 18.1,16.3 v18.4,16.3
  POWER 0.2: v24.2,5.7 24,5.7 23.9,5.8 22.5,7.2 22.5,7.6 22.5,7.8 22.5,9.6 | 22.5,9.6 22.5,9.8 21.2,11.1 20.9,11.4 v19.3,11.4 | v18.4,16.3 20,16.3 20.4,16.3 20.7,16 21.2,15.5 21.3,15.4 21.3,13.9 21.2,13.8 20.9,13.5 20.9,12.7 21,12.6 21.4,12.2 22.5,11.1 22.5,9.6
  Bottom 0.2: IC7.13 15.85,12.05 v16.1,12.3
+3V  (via drill 0.2, 0.25, 0.3)
  Top 0.2: R16.P$2 R15.P$2 v7.7,7.4 | IC9.7 13.75,6.85 v13.7,6.8 | LED.2 0.8,8.9 v0.8,8.6 | R30.P$2 21.9,20.4 v21.7,20.2 | C19.P$2 7.4,9.6 7.1,9.9 6.6,10.4 IC3.8
  Top 0.254: C1.P$2 21,13.55 IC4.1
  Top 0.305: C1.P$2 21,14.4 v20.7,14.7 | C19.P$2 C22.P$2 R18.P$2 10,9.2 v10.1,9.3 | R6.P$2 v16.8,5.7
  Top 0.406: IC3.8 6.6,13 7.85,14.25 12.2,14.25 13.8,12.65 IC3.17
  POWER 0.2: v7.7,7.4 7.6,7.4 7.4,7.6 7.4,8 9.2,9.8 9.2,10.2 | v13.7,6.8 13,6.1 13,6 | v16.8,18.1 15.7,17 15.7,16 16.6,15.1 16.6,15 | v0.8,8.6 1.6,7.8 6,7.8 7,8.8 7,9.9 9.2,12.1
  POWER 0.305: v20.7,14.7 19.6,14.7 19.5,14.8 19.3,15 19.1,15 16.6,15 15.3,15 15.2,15 10.5,15 9.3,13.8 9.2,13.7 9.2,12.1 9.2,10.2 9.2,9.7 | v16.8,5.7 16.6,5.5 15.8,5.5 15.3,6 13,6 12.8,6 10.6,6 10.5,6.1 9.2,7.4 9.2,7.9 9.2,8.7 9.2,9 9.2,9.7 | 9.2,9.7 9.4,9.5 9.9,9.5 v10.1,9.3
  Bottom 0.2: J3.4 16.93,18.8 | 16.93,18.8 16.93,18.23 v16.8,18.1 | 16.93,18.8 17.53,19.4 20.6,19.4 20.9,19.4 21.4,19.9 v21.7,20.2
+3V0_IMP  (via drill 0.2)
  Top 0.2: IC10.9 9.82,1.02 10,1.2 10.05,1.2 C18.P$2 10.45,1.6 IC5.1 | L2.P$2 12.2,4.9
  Top 0.305: 12.2,4.9 v11.6,4.9 | v10.7,2.2 10.7,1.95 IC5.1
  POWER 0.406: v10.7,2.2 10.7,3.9 10.7,4 v11.6,4.9
+3V3  (via drill 0.2)
  Top 0.2: 26.4,6.8 C2.P$1 26.1,6.9 24.6,6.9 23.95,6.25 IC6.1 22.7,6.4 v21.9,7.2 | v16.1,10.9 16.1,10.2 16.3,10 C13.P$2 16.8,10.2 16.7,10.2 v16.7,10.5
  POWER 0.2: v21.9,7.2 21.3,7.2 20.7,7.2 20.3,7.6 18.1,7.6 17.8,7.9 17.8,10.6 17.5,10.9 16.9,10.9 16.7,10.7 v16.7,10.5
  Bottom 0.2: IC7.15 15.95,11.05 v16.1,10.9
AD5933_VIN
  Top 0.2: IC10.5 3.08,2.98 6.6,6.5 R13.P$1 R12.P$2
AGND
  Top 0.2: IC10.14 IC10.13 8.88,3.6 9.7,3.6 10,3.9 10.3,3.9 C21.P$1 | IC8.4 15.72,0.82 16,1.1 16.5,1.6 16.5,2.4 16.5,2.7 16.4,2.7 | R4.P$2 21.3,2.1 21,2.4 20.8,2.4 19.8,3.4 17.7,3.4 17.6,3.4 16.9,2.7 16.4,2.7 | 15.6,3.3 15.65,3.25 | 15.65,3.25 16.2,2.7 16.4,2.7 | 15.65,3.25 15.4,3.5 15.4,3.9 15.3,4 15,4.3 14.7,4.3 14.4,4.3 R26.P$1 R11.P$2 13.2,4.9 12.9,5.2 12.7,5.4 12.3,5.4 11.3,5.4 11.1,5.2 10.6,4.7 C21.P$1 | C21.P$1 C20.P$1
ANALOG_+3V  (via drill 0.2)
  Top 0.2: v17.8,2.8 17.9,2.8 19,2.8 IC8.8 19.82,2.77 20.4,2.2 R3.P$1 | v13,2.9 12.7,2.9 12.6,2.9 R10.P$1
  Top 0.254: IC10.10 IC10.11
  Top 0.305: L2.P$1 R10.P$1 C20.P$2 C21.P$2 10.2,2.8 10.2,2.5 10.03,2.33 IC10.11
  POWER 0.2: v17.8,2.8 13.2,2.8 13.1,2.8 v13,2.9
BATT  (via drill 0.2, 0.25, 0.3, 0.35)
  Top 0.2: IC6.5 25.7,5.3 C8.P$1 26.5,4.5 v26.5,4 | R24.P$1 19.8,4 19.9,3.9 20.3,3.9 R1.P$1 | v24.2,3.5 24.3,3.4 24.3,1.1 24.55,0.85 IC2.P$4 25.4,0.6 R8.P$2 26.4,0.5 26.9,0.5 27.1,0.7 v27.1,1 | C5.P$2 21,12.64 IC4.4 | IC5.4 11.76,1.75 11.5,2 v11.5,2.2
  Top 0.305: IC4.4 21.14,12.74 v21.4,13 | J1.2 18.4,15.4 19.3,16.3 20,17 v20.2,17 | v17.7,4.7 17.2,4.7 C4.P$2 17,5 17.4,5.4 18.07,5.4 IC1.3 19.14,5.36 v19.4,5.1
  Top 0.406: R24.P$1 18.9,4.57 IC1.3
  POWER 0.2: v26.5,4 25.9,4
  POWER 0.305: v21.4,13 21.7,13.3 21.8,13.4 21.8,13.8 21.8,15.6 21.65,15.75 | 20.95,16.45 21.3,16.1 21.65,15.75 | 20.95,16.45 20.9,16.5 | 21.65,15.75 21.7,15.7 23.1,14.3 23.1,8.5 23.1,7.8 24.6,6.3 25.8,5.1 25.9,5 25.9,4 25.4,3.5 v24.2,3.5 21.3,3.5 21,3.5 v19.4,5.1 | 20.95,16.45 20.4,17 v20.2,17 | v11.5,2.2 11.5,2.8 12.9,4.2 17.2,4.2 v17.7,4.7
BLE_EN_1V8  (via drill 0.2)
  Top 0.2: R17.P$2 v21.5,8.4 | v24.2,4.9 24.2,4.7 24.55,4.35 IC6.4 | v16.5,13.4 16.2,13.1 IC3.19
  Bottom 0.2: v16.5,13.4 17,13.9 17,14.5 17.8,15.3 19.1,15.3 19.9,16.1 20.4,16.1 20.8,16.5 23,16.5 24.8,16.5 25.1,16.2 25.1,13.6 23.3,11.8 21.3,9.8 20.9,9.4 20.9,9 v21.5,8.4 22.7,8.4 24.8,6.3 24.8,5.5 v24.2,4.9
BLE_EN_3V3  (via drill 0.2)
  Top 0.2: v23.7,4.3 22.75,4.3 IC6.3 | IC3.20 16.2,13.9 v16.5,14.2 | R2.P$2 21.1,9.2 v21.5,9.2
  Bottom 0.2: v21.5,9.2 24.5,9.2 24.6,9.2 24.8,9 25.3,8.5 25.6,8.2 25.6,7.5 | v23.7,4.3 24.4,4.3 25.15,5.05 | 25.15,5.05 25.3,5.2 | v16.5,14.2 16.5,15.1 16.5,15.2 16.5,15.4 18.9,17.8 19.7,17.8 | 19.2,17.8 19.7,17.8 | 19.7,17.8 23,17.8 24.3,17.8 25.6,16.5 25.6,7.5 | 25.6,7.5 25.6,5.5 25.15,5.05
BLE_EN_IMP_3V0  (via drill 0.2)
  Top 0.2: IC3.27 v13,17.4 | v12.3,0.5 11.86,0.5 IC5.3
  Bottom 0.2: v12.3,0.5 24.1,0.5 27.2,3.6 27.2,6.1 26.6,6.7 26.6,17 24.8,18.8 23.8,18.8 18.2,18.8 18.1,18.9 17.7,18.9 17.4,18.6 17.4,17.9 16.8,17.3 16.5,17 13.4,17 v13,17.4
BLE_MAX_INT  (via drill 0.2)
  Top 0.2: R18.P$1 9.7,8.2 9.9,8.2 10.5,8.8 11,9.3 11,9.9 v11.1,10 10.6,10.5 IC3.13
  Bottom 0.2: IC7.7 12.45,11.05 12.25,11.05 12.15,11.05 v11.1,10
BLE_PROG_SWCLK  (via drill 0.2)
  Top 0.2: IC3.10 8.2,11.8 v8.2,12.8
  Bottom 0.2: v8.2,12.8 8.2,13.01 8.2,13.4 12,17.2 12,18.6 12.8,19.4 13.37,19.4 J3.2
BLE_PROG_SWDIO  (via drill 0.2)
  Top 0.2: IC3.9 7.4,10.2 7.7,9.9 v7.9,9.9
  Bottom 0.2: v7.9,9.9 8.1,9.9 8.2,10 8.2,11.8 8.3,11.9 8.5,12.1 8.7,12.3 9,12.6 9.5,13.1 9.5,14 12.4,16.9 12.4,17.8 13.8,19.2 14.44,19.2 J3.3
BLE_RESET  (via drill 0.2)
  Top 0.2: R31.P$2 v26.4,20.4 | IC3.34 7.4,19.8 v7.7,20.1
  POWER 0.2: v26.4,20.4 26.2,20.6 23.7,20.6 22.5,19.4 14.14,19.4 J3.1 12.94,20.6 11.4,20.6 8.4,20.6 8.2,20.6 v7.7,20.1
BLE_RESET_STS_INSERT  (via drill 0.2)
  Top 0.2: R30.P$1 23.8,20.4 v24.1,20.1 | R31.P$1 24.4,20.4 v24.1,20.1 | J2.1 24.9,18.7 24.1,19.5 v24.1,20.1 | IC3.29 v11.4,20.1
  POWER 0.2: v24.1,20.1 24.1,19.5 23.5,18.9 12.5,18.9 11.7,19.7 11.7,20.1 11.6,20.2 11.5,20.2 v11.4,20.1
BLE_SCL
  Top 0.2: IC10.16 9.3,6.03 R16.P$1 9.4,6.4 9.9,6.9 9.9,7.4 9.95,7.45 10,7.5 10.3,7.8 | IC9.1 10.95,7.35 10.75,7.35 10.3,7.8 | IC3.14 11.4,10.5 11.7,10.2 11.7,9.6 11.6,9.5 11.4,9.3 11.4,9.1 10.6,8.3 10.6,8.1 10.3,7.8
BLE_SDA  (via drill 0.2)
  Top 0.2: 8.82,4.9 IC10.15 7.78,4.92 7.4,5.3 7.4,6 v7.6,6.2 7.8,6.4 R15.P$1 | IC9.8 15.2,7.85 15.2,9 14.7,9.5 14.1,9.5 14,9.6 13.9,9.7 v13.8,9.7 12.9,9.7 12.2,10.4 IC3.15
  Bottom 0.2: v13.8,9.7 13.7,9.8 13.7,12 13.7,12.2 13.7,12.3 13.47,12.53 12.28,12.53 10.32,12.53 8.6,10.8 8.6,7.7 8.6,7.2 8.4,7 v7.6,6.2
BLE_STS_CHARGE  (via drill 0.2)
  Top 0.2: IC1.1 16.96,7.24 R6.P$1 | 18.14,7.2 IC1.1 | v21.6,6.6 19.9,6.6 19.26,7.24 IC1.1 | v17.9,18.2 16.8,17.1 IC3.24
  Bottom 0.2: v21.6,6.6 21.95,6.25 21.95,6.05 22.8,5.2 22.8,3.8 23.8,2.8 24.7,2.8 25.8,3.9 25.8,4.8 26.1,5.1 26.1,16.7 24.5,18.3 18,18.3 v17.9,18.2
BLE_UART_RX
  Top 0.2: J3.7 20,19.68 20,19.2 20,18.9 19.7,18.6 16.6,15.5 16.6,15.1 16.2,14.7 IC3.21
BLE_UART_TX
  Top 0.2: J3.6 19.4,20.35 19.4,19.3 19.4,18.9 18.8,18.3 16,15.5 IC3.22
BLE_VBATT_SENSE  (via drill 0.2)
  Top 0.2: R24.P$2 R25.P$1 17,3.6 v16.7,3.3 | IC3.12 9.8,10.3 v10,10.1
  Bottom 0.2: v10,10.1 10.2,10.1 10.7,9.6 10.8,9.5 10.8,8.7 10.6,8.5 10.6,8.3 10.6,6.6 11.4,5.8 15.8,5.8 16.1,5.5 16.1,3.6 16.4,3.3 v16.7,3.3
ECG_+
  Top 0.2: J2.3 22.8,13.6 21.6,12.4 21.6,11.4 21.4,11.2 R22.P$2
ECG_-
  Top 0.254: R21.P$2 24.14,10.3 J2.4
GND  (via drill 0.2, 0.25, 0.3, 0.35)
  Top 0.2: C8.P$2 C7.P$2 C2.P$2 v27.4,7.3 | R9.P$1 v27.2,1.7 | 7.5,0.4 v7.2,0.7 7.5,0.4 | v0.5,10 1,10.5 IC3.1 IC3.2 | C15.P$1 C14.P$1 18.2,13.9 18.2,14 v17.8,14.4 | IC2.P$2 v23.4,1.8 | C3.P$1 21.5,4.7 22,5.2 22.6,5.2 IC6.2 v23.7,5.3 | IC9.2 12.55,6.85 v12.6,6.8 | R17.P$1 R2.P$1 R5.P$2 19,9.3 18.8,9.3 v18.4,9.7 18.1,10 17.9,10 C13.P$1 | R23.P$1 19.3,14.3 19.6,14.6 | C5.P$1 19.9,12 v19.5,12 | C19.P$1 7.2,8 7.2,7.3 7.2,7 v7.3,6.9 | IC3.18 14.6,10.4 v14.3,10.1 | C1.P$1 20,13.55 IC4.2 20.25,13.1 IC4.5 | IC3.3 v2.6,10 | IC3.5 4.2,10.4 v4.6,10 | IC3.4 3.4,10.2 v3.6,10 | IC3.6 5,10.5 v5.4,10.1 5.8,10.5 IC3.7 | R26.P$2 v14.8,3.6 | R25.P$2 C4.P$1 | IC3.36 5.8,19.8 v6.1,20.1 | 7.5,0.4 10,0.4 10.15,0.55 C18.P$1 10.45,0.6 IC5.2 11.4,0.95 IC5.5 | IC10.12 7.88,2.98 v7.3,2.4
  Top 0.254: IC3.18 14.68,11.5 | v15.1,5.1 15.3,4.9 C4.P$1
  Top 0.305: 22.78,8.52 J2.5 26.18,8.52 v27.4,7.3 | C1.P$1 20,14.2 19.6,14.6 J1.1 | C22.P$1 C19.P$1 | IC3.25 15.07,18.3 v16.1,18.3
  Top 0.406: J1.1 20.23,15.23 v20.4,15.4 | IC1.2 19.1,6.3 v19.3,6.1
  Bottom 0.2: v14.3,10.1 14.35,10.05 IC7.17 IC7.16
  pour GND (isolate 0.305): 5.75,21 5.75,12 0,12 0,0 28,0 28,21
  pour Bottom (isolate 0.305): 0,12 5.75,12 5.75,21 28,21 28,0 0,0
  pour Top (isolate 0.305): 0,12 5.75,12 5.75,21 28,21 28,0 0,0
  pour POWER (isolate 0.305): 0,12 5.75,12 5.75,21 28,21 28,0 0,0
GNDA  (via drill 0.2)
  Top 0.2: C12.P$1 16.2,9.1 16.1,9.2 v16.1,9.5 | C10.P$2 C9.P$1 v14.1,9 | C17.P$1 C16.P$1 18,12.2 v18.5,12.2 18.8,12.5 18.8,13 19.1,13.3 R23.P$2
  Bottom 0.2: v14.1,9 14.1,9.2 14.3,9.4 14.45,9.55 IC7.18 16.05,9.55 v16.1,9.5 16.1,9.7 16.3,9.9 17,9.9 17.8,10.7 C16.P$1 18,12.2 v18.5,12.2
LED_BLUE  (via drill 0.2)
  Top 0.2: R28.P$1 3.9,8.9 3.7,9.1 3.7,9.3 v3.6,9.4 | IC3.32 9,19.8 v9.3,20.1
  Bottom 0.2: v3.6,9.4 3.4,9.4 3.1,9.7 3.1,10.3 4.1,11.3 4.2,11.4 6,11.4 6.3,11.7 7.2,12.6 7.2,13.5 7.2,13.7 9,15.5 9.6,16.1 9.6,18.1 9.6,19.8 v9.3,20.1
LED_GREEN  (via drill 0.2)
  Top 0.2: R27.P$2 3.1,9 v2.7,9.4 | IC3.33 8.2,19.8 v8.5,20.1
  Bottom 0.2: v2.7,9.4 2.1,9.4 2,9.5 2,10.4 2,10.5 2.1,10.6 2.3,10.8 2.7,10.8 3,10.8 4,11.8 5.8,11.8 6.1,12.1 6.8,12.8 6.8,13.8 6.8,13.9 8.2,15.3 8.9,16 8.9,18.4 8.9,19 8.9,19.7 v8.5,20.1
LED_RED  (via drill 0.2)
  Top 0.2: R29.P$1 4.7,8.9 4.3,9.3 v4.3,9.4 | IC3.28 v12.2,20.1
  Bottom 0.2: v4.3,9.4 4.1,9.6 4.1,10.6 4.5,11 6.2,11 7.6,12.4 7.6,13.5 10.4,16.3 10.4,20.3 10.7,20.6 12,20.6 12.2,20.4 v12.2,20.1
MAX_SCL  (via drill 0.2)
  Top 0.2: IC9.4 10.75,5.85 R20.P$1 10.5,5.3 v10.2,5
  Bottom 0.2: IC7.9 10.45,12.05 9,10.6 9,5.5 9.5,5 v10.2,5
MAX_SDA  (via drill 0.2)
  Top 0.2: R19.P$1 15.95,5.85 IC9.5 14.15,5.3 v14.1,5.3
  Bottom 0.2: IC7.8 10.55,11.55 9.5,10.5 9.4,10.4 9.4,7.1 10.8,5.7 11.1,5.4 13.4,5.4 13.5,5.3 v14.1,5.3
N$1  (via drill 0.2)
  Top 0.2: C9.P$2 v11.9,9 11.1,8.2 v11.1,7.9 | R21.P$1 19.6,10.3 v19.5,10.2
  Bottom 0.2: IC7.4 12.15,9.55 12.1,9.5 12,9.4 11.9,9.3 v11.9,9 | 11.25,6.55 11.5,6.3 12.4,6.3 18.3,6.3 18.9,6.9 19.3,6.9 19.5,7.1 19.5,7.5 19.5,9 19.5,10 v19.5,10.2 | 11.25,6.55 11.15,6.65 | v11.1,7.9 11.1,6.7 11.25,6.55
N$2  (via drill 0.2)
  Top 0.2: C11.P$2 v18.4,8.2
  Bottom 0.2: IC7.21 15.6,8 15.8,7.8 15.9,7.7 18.2,7.7 18.5,7.7 18.5,8.1 v18.4,8.2
N$3  (via drill 0.2)
  Top 0.2: v11.8,8.1 11.9,8.2 12.4,8.2 C10.P$1 | v19.3,10.8 19.4,10.8 19.5,10.8 19.9,11.2 R22.P$1
  Bottom 0.2: IC7.5 12.05,10.05 11.7,9.7 11.6,9.6 11.4,9.4 11.4,8.5 v11.8,8.1 11.8,7.4 11.9,7.3 12.1,7.3 12.5,7.3 12.6,7.3 13.5,7.3 14.1,7.3 18.8,7.3 19.1,7.6 19.1,9.7 19.1,9.8 18.8,10.1 18.8,10.6 19,10.8 v19.3,10.8
N$4
  Top 0.2: IC8.5 20.38,0.82 R3.P$2 R4.P$1
N$5  (via drill 0.2, 0.4)
  Top 0.2: v17.7,2.1 18.1,2.1 19,2.1 IC8.7 | R12.P$1 R7.P$1 5.6,9.3 5.6,9.5 5.5,9.6 5.1,9.6 v5,9.5 | v4.1,3.2 5,3.2 5.5,3.7 v6.1,3.7
  Bottom 0.2: 17.3,2.1 v17.7,2.1 16.9,2.1 16.6,1.8 13.6,1.8 13.3,1.8 11.6,3.5 11.4,3.5 7.5,3.5 7.3,3.7 v6.1,3.7 | v5,9.5 4.9,9.4 4.9,9.1 4.9,9 4.7,8.8 3.95,8.05 3.15,8.05 3.1,8 2.9,7.8 2.3,7.2 2.3,4.1 3.2,3.2 v4.1,3.2
N$6  (via drill 0.2, 0.4)
  Top 0.2: IC8.6 17.77,1.48 17.27,1.48 v17.2,1.4 | R7.P$2 6.6,9.5 v6.4,9.7
  Bottom 0.2: J5.1 J5.2 21.2,14.2 20.8,13.8 20.8,9.9 20.5,9.6 20.5,4.7 21.3,3.9 21.8,3.4 21.8,2.4 20.4,1 17.4,1 17.2,1.2 v17.2,1.4 16.3,1.4 13.5,1.4 13.1,1.4 11.4,3.1 11.2,3.1 8.6,3.1 7.2,3.1 6.7,2.6 v5.9,2.6 5.5,2.6 4.9,3.2 4.3,3.8 3.8,3.8 2.8,4.8 2.8,7 3.3,7.5 3.4,7.5 4.1,7.5 5.4,8.8 5.4,9.1 5.5,9.2 6,9.7 v6.4,9.7
N$7  (via drill 0.2)
  Top 0.2: C11.P$1 16.2,8.2 v16.1,8.3
  Bottom 0.2: IC7.20 15.85,8.55 v16.1,8.3
N$8  (via drill 0.2)
  Top 0.2: IC10.6 3.58,2.33 3.67,2.33 v4.3,1.7 | C6.P$2 13.2,0.9 13.1,1 12.5,1 v12.3,1.2
  Bottom 0.2: v4.3,1.7 11.8,1.7 v12.3,1.2
N$9
  Top 0.2: R5.P$1 19.1,8.2 19.9,7.4 20.54,7.4 IC1.5
N$10
  Top 0.2: R11.P$1 13.5,3.3 13.5,3.1 13.5,2.4 13.5,2.1 C6.P$1 | R10.P$2 13,2.2 C6.P$1 | IC8.3 13.72,1.48 C6.P$1
N$11
  Top 0.2: R14.P$2 R8.P$1 25.35,1.6 IC2.P$5
N$12  (via drill 0.2)
  Top 0.2: C12.P$2 18.3,9.1 18.4,9 v18.4,8.9
  Bottom 0.2: IC7.19 15.2,9 15.9,9 16,9 16.2,8.8 16.4,8.8 16.6,8.8 17.3,8.8 17.4,8.7 18.2,8.7 v18.4,8.9
N$13
  Top 0.2: IC2.P$6 25.15,2.85 25.6,3.3 R14.P$1 R9.P$2
N$14  (via drill 0.2)
  Top 0.2: 15.2,2.8 14.6,2.8 IC8.1 IC8.2 14.75,2.3 v15.7,2.3
  Bottom 0.2: v15.7,2.3 15.9,2.5 15.9,2.9 15.4,3.4 15.4,4 15,4.4 12.7,4.4 12.4,4.1 11.7,4.1 11.5,4.1 11.4,4.1 7.7,4.1 6.6,5.2 J4.1 J4.2
N$15  (via drill 0.2)
  Top 0.2: L1.P$1 18.5,10.6 17.9,10.6 17.4,10.6 16.9,11.1 16.9,11.2 C17.P$2 C16.P$2 16.7,12 16.4,11.7 16.2,11.7 v16.1,11.6
  Bottom 0.2: IC7.14 15.2,11.6 v16.1,11.6
N$16
  Top 0.2: IC10.4 3.02,3.62 5.6,6.2 R13.P$2
N$17
  Top 0.2: R29.P$2 4.7,7.2 4.1,6.6 LED.1
N$18
  Top 0.2: LED.4 2,7.7 2.7,7 3.7,7 3.9,7.2 R28.P$2
N$19
  Top 0.2: LED.3 2.25,8.5 2.65,8.1 3.05,7.7 R27.P$1
PWR_EN  (via drill 0.2)
  Top 0.2: IC2.P$1 21.75,2.75 21.5,3 | 21.5,3 R1.P$2 | IC4.3 19.55,12.74 v19.4,12.6 | 21.5,3 21.4,2.9 v21.1,2.9
  Bottom 0.2: v19.4,12.6 20.1,12.6 20.4,12.3 20.4,10.1 20,9.7 20,3.9 21,2.9 v21.1,2.9
VIN  (via drill 0.3)
  Top 0.305: IC1.4 20.76,5.36 20.8,5.4 21.2,5.8 v21.2,6 | J2.2 22.16,16.14 21.66,16.14 21.4,16.4 v21.4,17.2
  Top 0.406: C3.P$2 20.5,5.17 IC1.4
  POWER 0.305: v21.2,6 20.1,7.1 19.8,7.1 18.9,7.1 18.4,6.6 18.4,4 20.2,2.2 22,2.2 22.6,2.8 26.7,2.8 27.2,3.3 27.2,6 26.7,6.5 23.8,9.4 23.8,17.3 23.2,17.9 22.1,17.9 v21.4,17.2

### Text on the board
tPlace: v1.1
